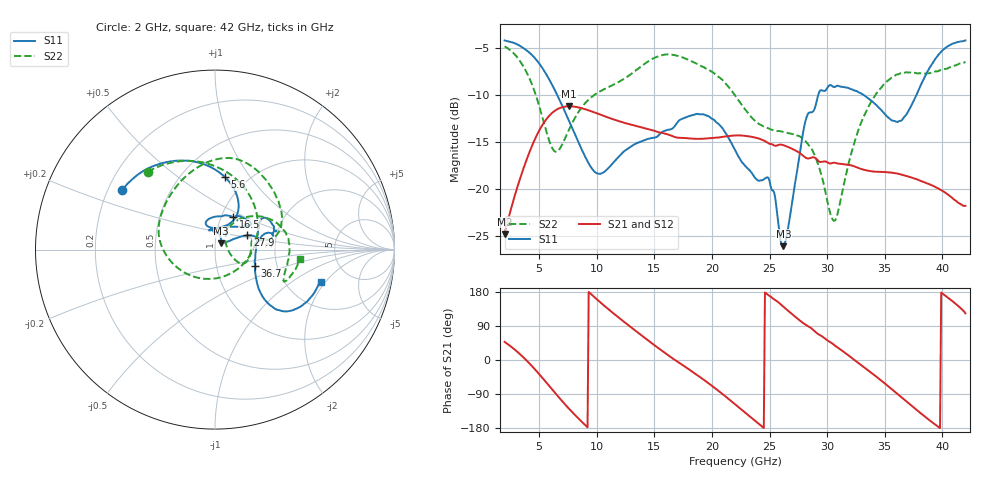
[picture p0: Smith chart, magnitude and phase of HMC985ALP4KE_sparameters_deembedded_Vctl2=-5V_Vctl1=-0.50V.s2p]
!s2p File: Measurements: S11, S21, S12, S22
# GHz S dB R 50.0
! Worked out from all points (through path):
!   401 points, 2 GHz to 42 GHz, reference 50 ohm
!   highest |S21| = -11.23 dB at 7.6 GHz (marker M1); lowest = -24.8 dB at 2 GHz (marker M2)
!   lowest |S11| = -26.1 dB at 26.2 GHz (marker M3), VSWR 1.10, Z = 53.4 + j3.84 ohm
!   |S11| at or under -10 dB: 6.552 GHz to 29.23 GHz (22.68 GHz wide, 127 % of centre); 33.14 GHz to 37.76 GHz (4.623 GHz wide, 13 % of centre)
!   |S22| runs from -23.4 to -4.8 dB; largest |S21 - S12| = 0.00028
!   S11 on the Smith chart (normalised r, x): 2 GHz: 0.26, +0.28; 5.6 GHz: 0.79, +0.77; 16.5 GHz: 1.14, +0.43; 27.9 GHz: 1.42, +0.23; 36.7 GHz: 1.54, -0.30; 42 GHz: 3.08, -1.78
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2  -4.22 147.3  -24.84 47.9  -24.84 47.9  -4.84 130.8
3.6  -5.01 120.6  -17.99 7.8  -17.99 7.8  -6.93 85.6
5.6  -7.79 82.2  -12.65 -58.7  -12.66 -58.7  -13.80 -4.7
6.5  -9.87 67.4  -11.60 -91.2  -11.60 -91.2  -16.06 -73.3
7.6  -12.79 57.8  -11.23 -128.9  -11.24 -128.9  -13.69 -139.2
8.7  -15.85 61.5  -11.44 -163.1  -11.44 -163.1  -11.33 -172.5
10.1  -18.40 87.0  -12.02 157.7  -12.02 157.7  -9.76 164.8
11.9  -16.61 109.7  -12.81 112.0  -12.82 112.0  -8.65 140.5
15.4  -14.29 77.1  -14.01 30.3  -14.02 30.3  -5.88 86.8
16.5  -13.64 60.8  -14.37 6.0  -14.38 6.0  -5.74 73.6
19.4  -12.16 35.1  -14.68 -54.6  -14.68 -54.6  -7.16 35.4
22  -15.87 52.4  -14.34 -116.7  -14.35 -116.7  -10.06 10.8
24.9  -18.85 101.3  -15.17 171.1  -15.18 171.1  -13.60 12.6
26.2  -26.13 46.5  -15.38 140.5  -15.38 140.6  -13.97 -2.1
27.9  -14.11 23.8  -16.48 97.8  -16.48 97.9  -14.67 -23.4
28.7  -11.86 11.8  -16.68 81.8  -16.68 81.8  -15.87 -28.1
30.7  -9.16 19.7  -17.25 37.6  -17.25 37.6  -23.38 24.1
32.9  -9.84 33.1  -17.89 -12.3  -17.89 -12.3  -13.13 50.8
35.4  -12.52 10.7  -18.28 -71.8  -18.28 -71.7  -8.38 21.3
36.7  -12.36 -22.2  -18.59 -104.8  -18.60 -104.7  -7.66 5.1
39.6  -5.86 -42.4  -19.95 -175.4  -19.96 -175.3  -7.50 -24.7
42  -4.22 -17.0  -21.83 123.0  -21.85 123.0  -6.48 -6.2
